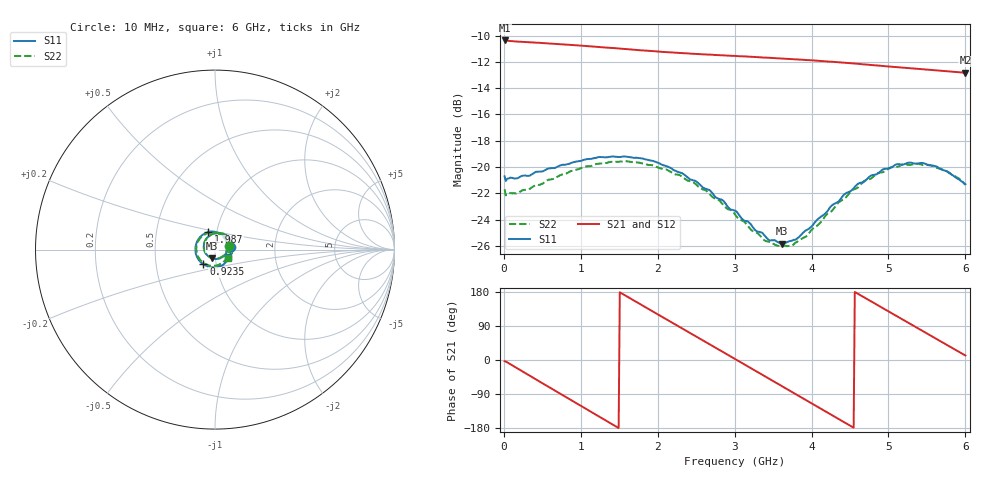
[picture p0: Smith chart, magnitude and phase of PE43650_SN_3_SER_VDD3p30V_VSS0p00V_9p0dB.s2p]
!Keysight Technologies,N5245B,MY57181451,A.13.50.07
!Date: Tuesday, May 07, 2019 08:00:02
!Correction: S11(Full 2 Port(1,2))
!S21(Full 2 Port(1,2))
!S12(Full 2 Port(1,2))
!S22(Full 2 Port(1,2))
!S2P File: Measurements: S11, S21, S12, S22:
# Hz S  dB  R 50
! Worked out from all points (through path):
!   401 points, 10 MHz to 6 GHz, reference 50 ohm
!   highest |S21| = -10.36 dB at 10 MHz (marker M1); lowest = -12.8 dB at 6 GHz (marker M2)
!   group delay of S21, straight-line fit = 327 ps
!   lowest |S11| = -25.8 dB at 3.619 GHz (marker M3), VSWR 1.11, Z = 48.1 - j4.65 ohm
!   |S11| at or under -10 dB: start of sweep to end of sweep
!   |S22| runs from -26.0 to -19.6 dB; largest |S21 - S12| = 0.0023
!   S11 on the Smith chart (normalised r, x): 10 MHz: 1.20, +0.04; 923.5 MHz: 0.87, -0.14; 1.987 GHz: 0.91, +0.18; 6 GHz: 1.16, -0.10
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1e7  -20.71 9.6  -10.36 -3.4  -10.42 -3.4  -21.69 12.7
2.496e8  -20.65 -37.2  -10.48 -30.9  -10.52 -31.0  -21.75 -37.4
5.1915e8  -20.29 -75.5  -10.57 -63.5  -10.62 -63.5  -21.21 -76.4
9.23475e8  -19.60 -128.2  -10.73 -112.0  -10.78 -112.0  -20.22 -128.2
1.013325e9  -19.51 -139.4  -10.77 -122.7  -10.82 -122.7  -20.05 -139.4
1.2679e9  -19.24 -169.3  -10.88 -153.0  -10.94 -153.0  -19.73 -168.6
1.492525e9  -19.23 164.8  -10.98 -179.6  -11.04 -179.6  -19.60 166.4
1.732125e9  -19.30 138.2  -11.09 152.1  -11.15 152.1  -19.65 140.6
1.9867e9  -19.64 110.7  -11.20 122.2  -11.26 122.2  -20.00 113.7
2.01665e9  -19.71 107.4  -11.21 118.6  -11.26 118.7  -20.06 110.5
2.241275e9  -20.32 82.6  -11.30 92.3  -11.35 92.3  -20.56 86.2
2.4659e9  -21.02 57.0  -11.38 66.0  -11.43 66.0  -21.16 62.0
2.750425e9  -22.28 24.0  -11.47 32.6  -11.52 32.7  -22.41 28.9
3.005e9  -23.33 -9.9  -11.54 2.7  -11.60 2.8  -23.60 -2.9
3.289525e9  -24.90 -52.3  -11.63 -30.7  -11.68 -30.6  -25.00 -45.4
3.618975e9  -25.84 -109.4  -11.74 -69.4  -11.79 -69.4  -26.00 -101.8
4.008325e9  -24.47 -176.8  -11.88 -115.2  -11.93 -115.3  -24.75 -169.3
4.277875e9  -22.86 145.0  -11.99 -147.0  -12.04 -147.0  -23.24 151.2
4.517475e9  -21.79 114.0  -12.10 -175.2  -12.15 -175.1  -21.81 120.3
5.01165e9  -20.10 59.8  -12.35 127.0  -12.40 127.1  -20.07 65.2
5.4609e9  -19.71 16.2  -12.56 74.6  -12.61 74.7  -19.85 19.8
6e9  -21.31 -30.6  -12.83 11.9  -12.87 11.9  -21.35 -31.5
